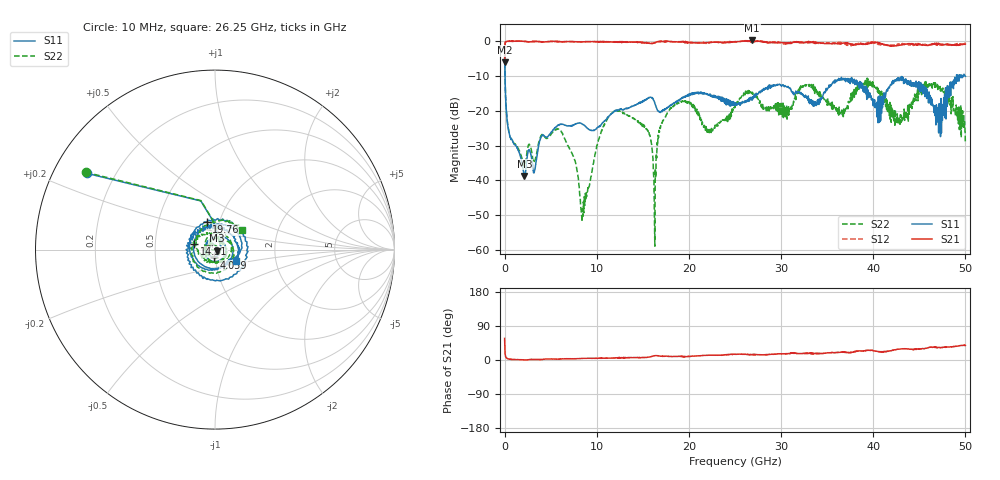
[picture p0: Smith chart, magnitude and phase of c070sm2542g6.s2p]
! 7/14/2021 1:26:38 PM
! D:\C070SM2542G6.S2P
! CHANNEL.1
! TR.MEASUREMENT
! CORRECTED.DATA
# GHZ S RI R 50.0
! FREQ.GHZ  S11RE  S11IM  S21RE  S21IM  S12RE  S12IM  S22RE  S22IM
!; PortSelection: Port_12
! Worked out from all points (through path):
!   1001 points, 10 MHz to 50 GHz, reference 50 ohm
!   highest |S21| = 0.18 dB at 26.85 GHz (marker M1); lowest = -6.1 dB at 10 MHz (marker M2)
!   lowest |S11| = -38.7 dB at 2.16 GHz (marker M3), VSWR 1.02, Z = 50.9 - j0.689 ohm
!   |S11| at or under -10 dB: 54.73 MHz to 49.04 GHz (48.99 GHz wide, 200 % of centre); 49.57045 GHz to 49.68759 GHz (117.1 MHz wide, 0.236 % of centre); 49.71966 GHz to 49.80605 GHz (86.39 MHz wide, 0.174 % of centre)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
!   |S22| runs from -58.9 to -1.6 dB; largest |S21 - S12| = 0.085
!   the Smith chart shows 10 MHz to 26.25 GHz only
!   S11 on the Smith chart (normalised r, x): 10 MHz: 0.10, +0.27; 4.059 GHz: 0.99, -0.09; 14.31 GHz: 0.79, +0.05; 19.76 GHz: 0.87, +0.28; 26.25 GHz: 1.25, -0.17
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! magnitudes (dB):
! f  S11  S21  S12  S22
! 10 MHz  -1.6  -6.1  -6.1  -1.6
! 509.9 MHz  -26.5  -0.1  -0.1  -26.5
! 2.16 GHz  -38.7  -0.1  -0.1  -36.0
! 4.059 GHz  -27.1  -0.2  -0.2  -26.8
! 6.259 GHz  -23.9  -0.1  -0.2  -26.5
! 8.358 GHz  -23.7  -0.2  -0.2  -49.8
! 11.26 GHz  -21.7  -0.2  -0.2  -21.9
! 14.31 GHz  -18.3  -0.4  -0.2  -22.7
! 15.71 GHz  -16.3  -0.6  -0.7  -26.9
! 16.26 GHz  -17.4  -0.5  -0.5  -49.6
! 16.71 GHz  -20.2  -0.2  -0.1  -27.8
! 19.76 GHz  -15.9  -0.5  -0.2  -17.2
! 22.16 GHz  -15.5  -0.4  -0.5  -25.8
! 25 GHz  -17.8  -0.1  -0.3  -19.1
! 26.25 GHz  -17.4  0.0  0.0  -14.6
! 26.85 GHz  -17.0  0.2  -0.2  -14.6
! 30.5 GHz  -13.0  -0.6  -0.6  -19.3
! 33.35 GHz  -17.0  -0.3  -0.4  -13.7
! 39.6 GHz  -15.9  -0.6  -0.4  -12.7
! 41.7 GHz  -13.2  -1.3  -1.1  -18.8
! 46.7 GHz  -21.4  -0.9  -0.9  -13.8
! 50 GHz  -10.1  -0.9  -0.8  -29.5
